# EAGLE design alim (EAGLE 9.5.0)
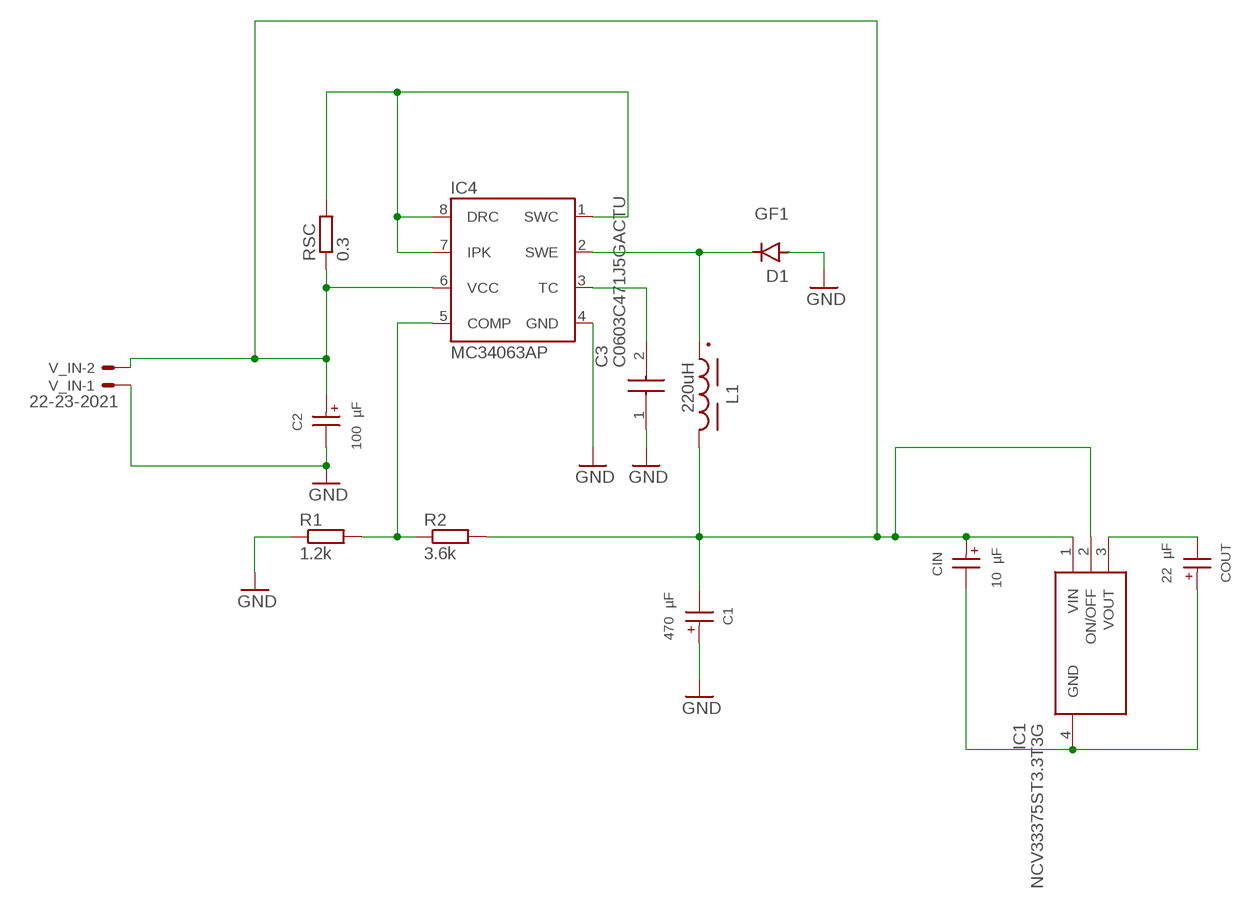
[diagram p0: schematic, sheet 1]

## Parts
C1  470 µF  WCAP-ASLL_8X10.5_865060353009  [WCAP-ASLL_8X10.5(DXL)]
C2  100 µF  WCAP-ASLL_6.3X7.7_865060445005  [WCAP-ASLL_6.3X7.7(DXL)]
C3  C0603C471J5GACTU  [C0603]
CIN  10 µF  WCAP-ASLL_4X5.5_865060440001  [WCAP-ASLL_4X5.5(DXL)]
COUT  22 µF  WCAP-ASLL_5X5.5_865060442002  [WCAP-ASLL_5X5.5(DXL)]
D1  GF1  [SMA-DO214AC]
IC1  NCV33375ST3.3T3G  [SOT230P700X175-4N]
IC4  MC34063AP  [DIL-08]
L1  220uH  WE-PDA_1260_784771221  [WE-PDA_1260]
R1  1.2k  R-EU_R0603  [R0603]
R2  3.6k  R-EU_R0603  [R0603]
RSC  0.3  R-EU_R1206W  [R1206W]
V_IN  22-23-2021  [22-23-2021]

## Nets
GND: C1.1(+) C2.2(-) C3.1 D1.A IC4.4(GND) R1.1 V_IN.1
N$1: IC4.5(COMP) R1.2 R2.1
N$3: C1.2(-) C2.1(+) CIN.1(+) IC1.1(VIN) IC1.2(ON/OFF) IC4.6(VCC) L1.2 R2.2 RSC.1 V_IN.2
N$4: COUT.2(-) IC1.3(VOUT)
N$5: CIN.2(-) COUT.1(+) IC1.4(GND)
N$6: D1.K(C) IC4.2(SWE) L1.1
N$7: C3.2 IC4.3(TC)
N$8: IC4.1(SWC) IC4.7(IPK) IC4.8(DRC) RSC.2

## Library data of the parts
C1 = c1:WCAP-ASLL_8X10.5: WCAP-ASLL Aluminium Electrolytic Capacitors; DATASHEET-URL: https://www.we-online.com/catalog/datasheet/865060353009.pdf; DF: 16%; DIAMETER: 8mm; I-LEAK: 75.2uA; I-RIPPLE: 600mA; L: 10.5mm; OPERATING-TEMPERATURE: -55 °C up to +105 °C; PART-NUMBER: 865060353009; TECHNICAL-REFERENCE: ASEE105471M016DVCTEE000; VR: 16V(DC); Z: 0.17Ohm
C2 = c2:WCAP-ASLL_6.3X7.7: WCAP-ASLL Aluminium Electrolytic Capacitors; DATASHEET-URL: https://www.we-online.com/catalog/datasheet/865060445005.pdf; DF: 14%; DIAMETER: 6.3mm; I-LEAK: 25uA; I-RIPPLE: 300mA; L: 7.7mm; OPERATING-TEMPERATURE: -55 °C up to +105 °C; PART-NUMBER: 865060445005; TECHNICAL-REFERENCE: ASED077101M025DVCTCB000; VR: 25V(DC); Z: 0.36Ohm
C3 = c3:C0603C471J5GACTU: SMD Comm C0G, Ceramic, 470 pF, 5%, 50 VDC, 125 VDC, 125?C, -55?C, C0G, SMD, MLCC, Ultra-Stable, Low Loss, Class I, 0.1 % , 100 GOhms, 3.7 mg, 0603, 1.6mm,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; ARROW_PART_NUMBER: C0603C471J5GACTU; ARROW_PRICE-STOCK: https://www.arrow.com/en/products/c0603c471j5gactu/kemet-corporation?region=nac; DESCRIPTION: SMD Comm C0G, Ceramic, 470 pF, 5%, 50 VDC, 125 VDC, 125?C, -55?C, C0G, SMD, MLCC, Ultra-Stable, Low Loss, Class I, 0.1 % , 100 GOhms, 3.7 mg, 0603, 1.6mm, 0.8mm, 0.8mm, 0.7mm, 0.35mm, 4000, 78 Weeks, 120; HEIGHT: 0.87mm; MANUFACTURER_NAME: KEMET; MANUFACTURER_PART_NUMBER: C0603C471J5GACTU; MOUSER_PART_NUMBER: 80-C0603C471J5G; MOUSER_PRICE-STOCK: https://www.mouser.co.uk/ProductDetail/KEMET/C0603C471J5GACTU?qs=6Zy9Yzz7FWCvDjERNKhvPg%3D%3D
CIN = cin:WCAP-ASLL_4X5.5: WCAP-ASLL Aluminium Electrolytic Capacitors; DATASHEET-URL: https://www.we-online.com/catalog/datasheet/865060440001.pdf; DF: 14%; DIAMETER: 4mm; I-LEAK: 3uA; I-RIPPLE: 90mA; L: 5.5mm; OPERATING-TEMPERATURE: -55 °C up to +105 °C; PART-NUMBER: 865060440001; TECHNICAL-REFERENCE: ASEB055100M025DVCTAB000; VR: 25V(DC); Z: 1.35Ohm
COUT = cout:WCAP-ASLL_5X5.5: WCAP-ASLL Aluminium Electrolytic Capacitors; DATASHEET-URL: https://www.we-online.com/catalog/datasheet/865060442002.pdf; DF: 14%; DIAMETER: 5mm; I-LEAK: 5.5uA; I-RIPPLE: 150mA; L: 5.5mm; OPERATING-TEMPERATURE: -55 °C up to +105 °C; PART-NUMBER: 865060442002; TECHNICAL-REFERENCE: ASEC055220M025DVCTBB000; VR: 25V(DC); Z: 0.8Ohm
D1 = diode:GF1: DIODE
IC1 = SamacSys_Parts:NCV33375ST3.3T3G: ON SEMICONDUCTOR - NCV33375ST3.3T3G - Fixed LDO Voltage Regulator, 4.3V to 13V, 260mV Dropout, 3.3Vout, 300mAout, SOT-223-4 Source: Datasheet; DESCRIPTION: ON SEMICONDUCTOR - NCV33375ST3.3T3G - Fixed LDO Voltage Regulator, 4.3V to 13V, 260mV Dropout, 3.3Vout, 300mAout, SOT-223-4; HEIGHT: 1.75mm; MANUFACTURER_NAME: onsemi; MANUFACTURER_PART_NUMBER: NCV33375ST3.3T3G; MOUSER_PART_NUMBER: 863-NCV33375ST3.3T3G; MOUSER_PRICE-STOCK: https://www.mouser.co.uk/ProductDetail/ON-Semiconductor/NCV33375ST33T3G?qs=Pqj8oIac8rWOl%252BM3OwXrOg%3D%3D
IC4 = v-reg-3:MC34063A: 1.5A Step-Up/Down/Inverting Switching Regulator NPN Darlington Switch, Vin 3V to 40V, Current Limiter Input, adjustable Frequency up to 100kHz
L1 = l:WE-PDA_1260: WE-PDA SMD Shielded Power Inductor; DATASHEET-URL: https://www.we-online.com/catalog/datasheet/784771221.pdf; FRES: 3.9MHz; IR: 0.99A; ISAT: 1.1A; MOUNT: SMT; PART-NUMBER: 784771221; RDC-MAX: 348mOhm; RDC-TYP: 290mOhm
R1 R2 RSC = rcl:R-EU_: RESISTOR, European symbol; SPICEPREFIX: R
V_IN = con-molex:22-23-2021: .100" (2.54mm) Center Header - 2 Pin; MF: MOLEX; MPN: 22-23-2021; OC_FARNELL: 1462926; OC_NEWARK: 25C3832

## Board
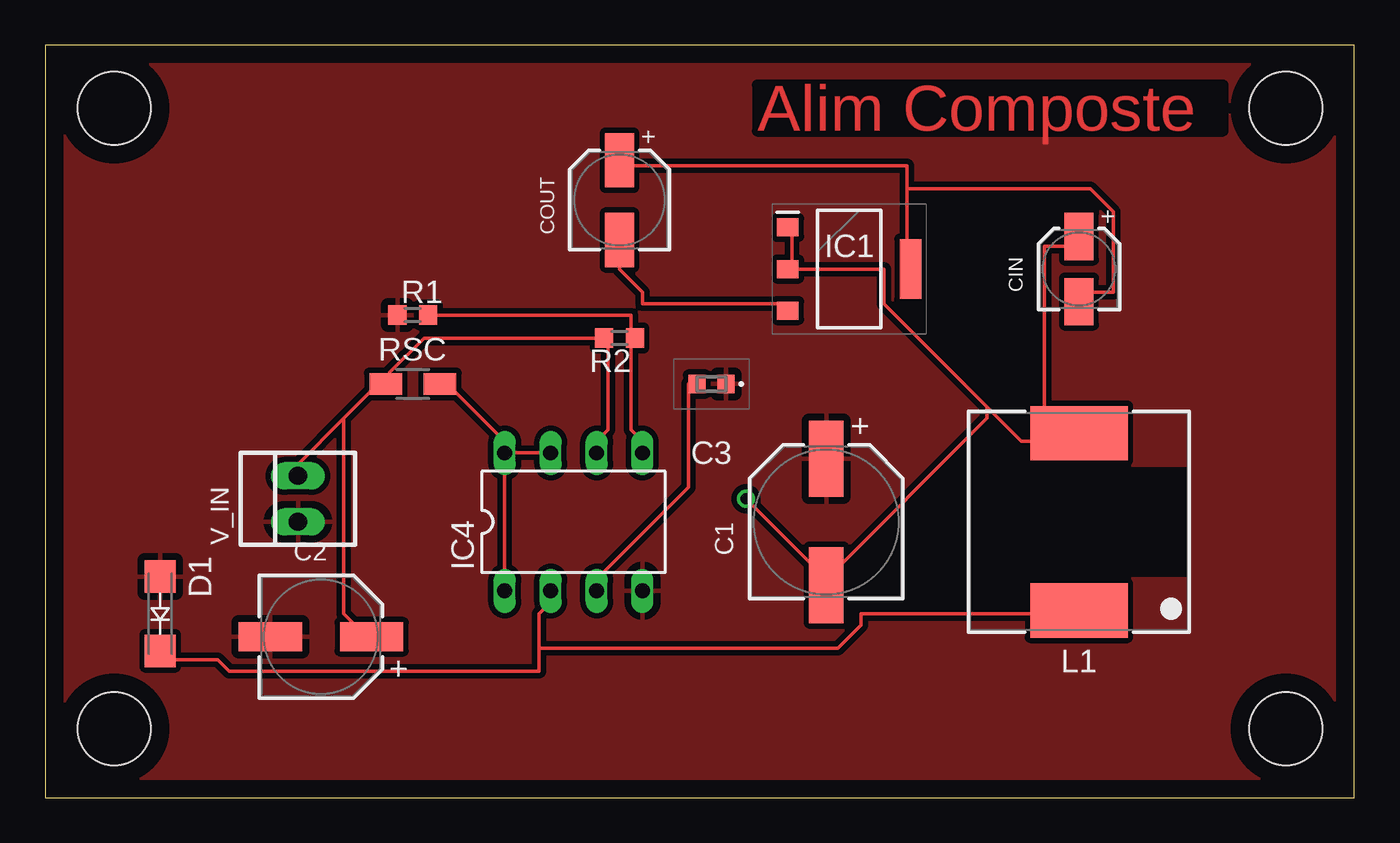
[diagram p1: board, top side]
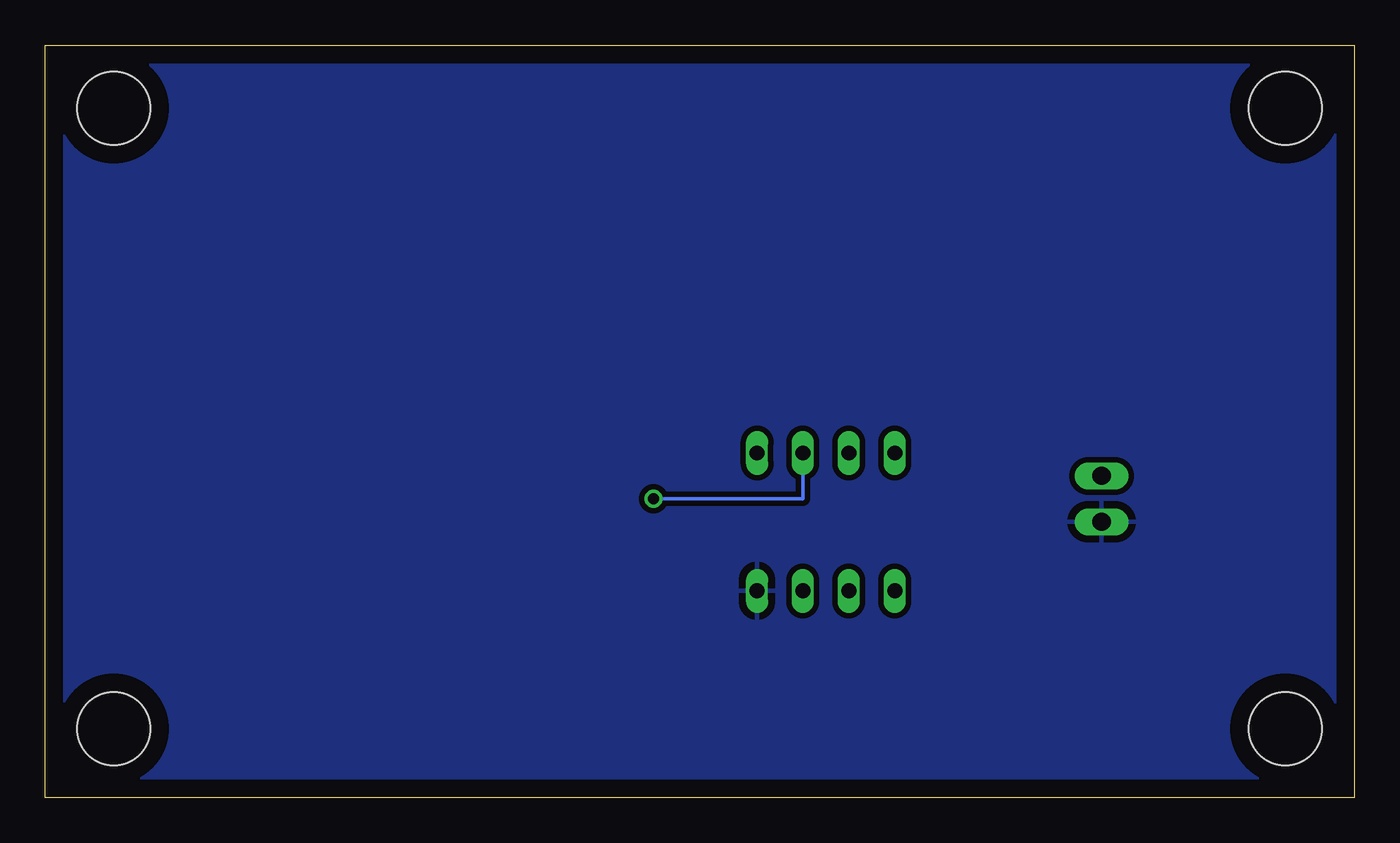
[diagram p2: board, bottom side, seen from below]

Size 72.37 x 41.58 mm. Coordinates in mm from the lower left corner, seen from the top.
Outline: 0,0 72.37,0 72.37,41.58 0,41.58 0,0
Copper layers (1*16): Top 0.035mm / dielectric 1.5mm / Bottom 0.035mm
Design rules "ENSEA_2022_04_08 *": minimum track width 0.2mm, minimum drill 0.6mm, track to track 0.3mm, track to pad 0.3mm, pad to pad 0.3mm, via to via 0.3mm, smd to smd 0.3mm, copper to edge 1mm, drill to drill 0.4mm, minimum pad ring 0.2mm, minimum via ring 0.2mm, stop-mask expansion 4mil, vias tented up to drill 0mil, thermal gap 0.4mm
Holes 4.06 mm at 68.58,3.81 68.58,38.1 3.81,38.1 3.81,3.81

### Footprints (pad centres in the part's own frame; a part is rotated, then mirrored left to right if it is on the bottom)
WCAP-ASLL_8X10.5(DXL) = smd 4.2 x 1.9: 1 3.5,0; 2 -3.5,0
WCAP-ASLL_6.3X7.7(DXL) = smd 3.5 x 1.6: 1 2.8,0; 2 -2.8,0
C0603 = smd 0.95 x 1: 1 -0.8,0; 2 0.8,0
WCAP-ASLL_4X5.5(DXL) = smd 2.6 x 1.6: 1 1.8,0; 2 -1.8,0
WCAP-ASLL_5X5.5(DXL) = smd 3 x 1.6: 1 2.2,0; 2 -2.2,0
SMA-DO214AC = smd 1.8 x 1.7: A -2.05,0; K 2.05,0
SOT230P700X175-4N = smd 1.2 x 1: 1 -3.4,2.3; 2 -3.4,0; 3 -3.4,-2.3 | smd 1.2 x 3.3: 4 3.4,0
DIL-08 = drill 0.813 long: 1 -3.81,-3.81; 2 -1.27,-3.81; 3 1.27,-3.81; 4 3.81,-3.81; 5 3.81,3.81; 6 1.27,3.81; 7 -1.27,3.81; 8 -3.81,3.81
WE-PDA_1260 = smd 5.4 x 3: 1 0,4.9; 2 0,-4.9
R0603 = smd 1 x 1.1: 1 -0.85,0; 2 0.85,0
R1206W = smd 1.8 x 1.2: 1 -1.499,0; 2 1.499,0
22-23-2021 = drill 1 long: 1 -1.27,0; 2 1.27,0

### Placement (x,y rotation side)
C1  43.18,15.24 90 top
C2  15.24,8.89 0 top
C3  36.83,22.86 180 top
CIN  57.15,29.21 90 top
COUT  31.75,33.02 90 top
D1  6.35,10.16 270 top
IC1  44.45,29.21 0 top
IC4  29.21,15.24 0 top
L1  57.15,15.24 180 top
R1  20.32,26.67 0 top
R2  31.75,25.4 180 top
RSC  20.32,22.86 0 top
V_IN  13.97,16.51 90 top

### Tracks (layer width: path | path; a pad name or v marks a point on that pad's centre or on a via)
GND
  pour Top: 0,40.64 0,0 72.39,0 72.39,41.91 0,41.91
  pour Bottom: 0,41.91 0,0 72.39,0 72.39,41.91
N$1
  Top 0.2: 32.38,25.4 32.38,20.32 33.02,19.68 IC4.5 | R1.2 32.38,26.67 32.38,25.4 | 32.38,25.4 R2.1
N$3  (via drill 0.6)
  Top 0.2: IC4.6 30.48,19.68 31.11,20.32 31.11,25.4 R2.2 20.95,25.4 19.05,23.49 19.05,22.86 RSC.1 18.41,22.86 16.51,20.95 | 16.51,20.95 13.97,18.41 V_IN.2 | 16.51,20.95 16.51,10.16 17.78,8.89 C2.1 | 41.28,29.21 41.28,31.11 IC1.1 | 41.28,29.21 46.36,29.21 46.36,27.3 52.07,21.59 | 52.07,21.59 53.98,19.68 55.25,19.68 | 55.25,19.68 57.15,19.68 L1.2 55.25,19.68 | 41.28,29.21 IC1.2 | 55.25,19.68 55.25,30.48 57.15,30.48 CIN.1 | 43.18,12.07 52.07,20.95 52.07,21.59 | 43.18,12.07 v38.74,16.51 | 43.18,12.07 C1.2
  Bottom 0.2: IC4.6 30.48,16.51 v38.74,16.51
N$4
  Top 0.2: COUT.2 31.75,29.21 33.02,27.94 33.02,27.3 40.64,27.3 IC1.3
N$5
  Top 0.2: 47.62,33.66 57.79,33.66 59.05,32.38 59.05,27.94 57.15,27.94 CIN.2 | 47.62,33.66 47.62,29.21 IC1.4 | 47.62,33.66 47.62,34.92 31.75,34.92 COUT.1
N$6
  Top 0.2: 27.3,8.25 27.3,10.16 27.94,10.8 IC4.2 | 27.3,8.25 27.3,6.99 10.16,6.99 9.53,7.62 6.35,7.62 D1.K | 27.3,8.25 43.82,8.25 45.09,9.53 45.09,10.16 57.15,10.16 L1.1
N$7
  Top 0.2: IC4.3 30.48,12.07 35.56,17.14 35.56,22.86 C3.2
N$8
  Top 0.2: IC4.8 25.4,19.68 22.22,22.86 RSC.2 | IC4.8 IC4.1 | IC4.8 IC4.7

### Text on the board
Top: Alim Composte

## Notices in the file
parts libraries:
l: Copyright: Würth Elektronik
